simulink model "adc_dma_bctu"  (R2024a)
settings: Solver=FixedStepAuto  StartTime=0.0  StopTime=10.0  FixedStep=0.001  RelTol=1e-3  EnableMultiTasking=on
PreLoadFcn:
  | % NXP_MBDT_S32K3 callback: DO NOT REMOVE
  | mbd_s32k3.common.nxp.model_callbacks.preLoadFcn();
PostLoadFcn:
  | % NXP_MBDT_S32K3 callback: DO NOT REMOVE
  | mbd_s32k3.common.nxp.model_callbacks.postLoadFcn();
InitFcn:
  | % NXP_MBDT_S32K3 callback: DO NOT REMOVE
  | mbd_s32k3.common.nxp.model_callbacks.initFcn();
libraries: mbd_s32k3_io_library x18, mbd_s32k3_isr_library x4, mbd_s32k3_cdd_library x4, mbd_s32k3_utility_library x1, simulink x1

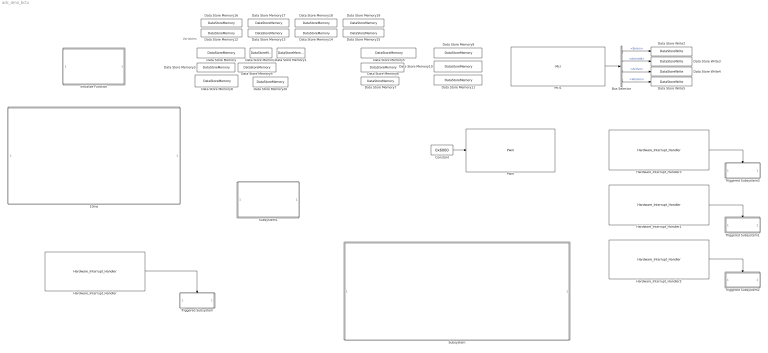
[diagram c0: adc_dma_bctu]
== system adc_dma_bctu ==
  note: Variables
  10ms : Subsystem  TreatAsAtomicUnit=on  SystemSampleTime=0.01
  Bus Selector : BusSelector  Commented=on  OutputSignals=Errors,ActiveId,Active,Version
  Constant : Constant  Commented=on  Value=0x6000
  Data Store Memory : DataStoreMemory  DataStoreName=Adc1_Group0_ResoultBuffer  WriteAfterWriteMsg=warning  ShowAdditionalParam=off  OutDataTypeStr=uint16
  Data Store Memory1 : DataStoreMemory  DataStoreName=GroupStatus  WriteAfterWriteMsg=warning  ShowAdditionalParam=off  OutDataTypeStr=uint32
  Data Store Memory10 : DataStoreMemory  DataStoreName=Bctu_NDataFlag  WriteAfterWriteMsg=warning  ShowAdditionalParam=off  OutDataTypeStr=boolean
  Data Store Memory11 : DataStoreMemory  DataStoreName=Bctu_OvrDataFlag  WriteAfterWriteMsg=warning  ShowAdditionalParam=off  OutDataTypeStr=boolean
  Data Store Memory12 : DataStoreMemory  DataStoreName=Errors_Instance  ReadBeforeWriteMsg=warning  WriteAfterWriteMsg=warning  WriteAfterReadMsg=warning  ShowAdditionalParam=off  OutDataTypeStr=uint32
  Data Store Memory13 : DataStoreMemory  DataStoreName=ActiveId_Instance  ReadBeforeWriteMsg=warning  WriteAfterWriteMsg=warning  WriteAfterReadMsg=warning  ShowAdditionalParam=off  OutDataTypeStr=uint8
  Data Store Memory14 : DataStoreMemory  DataStoreName=Active_Instance  ReadBeforeWriteMsg=warning  WriteAfterWriteMsg=warning  WriteAfterReadMsg=warning  ShowAdditionalParam=off  OutDataTypeStr=boolean
  Data Store Memory15 : DataStoreMemory  DataStoreName=Version_Instance  ReadBeforeWriteMsg=warning  WriteAfterWriteMsg=warning  WriteAfterReadMsg=warning  ShowAdditionalParam=off  OutDataTypeStr=uint8
  Data Store Memory16 : DataStoreMemory  DataStoreName=ChannelState  ReadBeforeWriteMsg=warning  WriteAfterWriteMsg=warning  WriteAfterReadMsg=warning  InitialValue=Mcl_DmaChannelStateType.MCL_DMA_CH_RESET_STATE  ShowAdditionalParam=off  OutDataTypeStr=Enum: Mcl_DmaChannelStateType
  Data Store Memory17 : DataStoreMemory  DataStoreName=Error_Channel  ReadBeforeWriteMsg=warning  WriteAfterWriteMsg=warning  WriteAfterReadMsg=warning  ShowAdditionalParam=off  OutDataTypeStr=uint32
  Data Store Memory18 : DataStoreMemory  DataStoreName=Active_Channel  ReadBeforeWriteMsg=warning  WriteAfterWriteMsg=warning  WriteAfterReadMsg=warning  ShowAdditionalParam=off  OutDataTypeStr=boolean
  Data Store Memory19 : DataStoreMemory  DataStoreName=Done_Channel  ReadBeforeWriteMsg=warning  WriteAfterWriteMsg=warning  WriteAfterReadMsg=warning  ShowAdditionalParam=off  OutDataTypeStr=boolean
  Data Store Memory2 : DataStoreMemory  DataStoreName=ADC_POT0  WriteAfterWriteMsg=warning  ShowAdditionalParam=off  OutDataTypeStr=uint16
  Data Store Memory20 : DataStoreMemory  DataStoreName=Adc1_ChansArray  WriteAfterWriteMsg=warning  ShowAdditionalParam=off  OutDataTypeStr=uint16
  Data Store Memory3 : DataStoreMemory  DataStoreName=Adc1_ReadStatus  WriteAfterWriteMsg=warning  ShowAdditionalParam=off  OutDataTypeStr=uint32
  Data Store Memory4 : DataStoreMemory  DataStoreName=Adc1_BufReadStatus  WriteAfterWriteMsg=warning  ShowAdditionalParam=off  OutDataTypeStr=uint32
  Data Store Memory5 : DataStoreMemory  DataStoreName=Adc0_Group0_ResoulBuffer  WriteAfterWriteMsg=warning  ShowAdditionalParam=off  OutDataTypeStr=uint16
  Data Store Memory6 : DataStoreMemory  DataStoreName=ADC_BCTU_Result  WriteAfterWriteMsg=warning  ShowAdditionalParam=off  OutDataTypeStr=uint16
  Data Store Memory7 : DataStoreMemory  DataStoreName=Adc0_ReadStatus  WriteAfterWriteMsg=warning  ShowAdditionalParam=off  OutDataTypeStr=uint32
  Data Store Memory8 : DataStoreMemory  DataStoreName=Calibration_ADC1_Status  WriteAfterWriteMsg=warning  ShowAdditionalParam=off  OutDataTypeStr=uint8
  Data Store Memory9 : DataStoreMemory  DataStoreName=Bctu_TriggerFlag  WriteAfterWriteMsg=warning  ShowAdditionalParam=off  OutDataTypeStr=boolean
  Data Store Write2 : DataStoreWrite  Commented=on  DataStoreName=Errors_Instance  IndexOptions=Index vector (dialog)  Indices=1  OutputSizes=1
  Data Store Write3 : DataStoreWrite  Commented=on  DataStoreName=ActiveId_Instance  IndexOptions=Index vector (dialog)  Indices=1  OutputSizes=1
  Data Store Write4 : DataStoreWrite  Commented=on  DataStoreName=Active_Instance  IndexOptions=Index vector (dialog)  Indices=1  OutputSizes=1
  Data Store Write5 : DataStoreWrite  Commented=on  DataStoreName=Version_Instance  IndexOptions=Index vector (dialog)  Indices=1  OutputSizes=1
  Hardware_Interrupt_Handler : mbd_s32k3_isr_library/Hardware_Interrupt_Handler  Priority=2  blockCbk=0  irqGroup=Adc  irqHandlers=Adc_Adc1Group0_Callback  irqSim=off  text=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
  Hardware_Interrupt_Handler1 : mbd_s32k3_isr_library/Hardware_Interrupt_Handler  Priority=2  Commented=on  blockCbk=0  irqGroup=Adc  irqHandlers=Bctu_NewData_Cb  irqSim=off  text=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
  Hardware_Interrupt_Handler2 : mbd_s32k3_isr_library/Hardware_Interrupt_Handler  Priority=2  Commented=on  blockCbk=0  irqGroup=Adc  irqHandlers=Bctu_OverrunData_Cb  irqSim=off  text=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
  Hardware_Interrupt_Handler3 : mbd_s32k3_isr_library/Hardware_Interrupt_Handler  Priority=2  Commented=on  blockCbk=0  irqGroup=Adc  irqHandlers=Bctu_Trg_Cb  irqSim=off  text=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
  Initialize Function : Subsystem  TreatAsAtomicUnit=on
  Mcl1 : mbd_s32k3_cdd_library/Mcl  Commented=on  api_func=Mcl_GetDmaInstanceStatus  logicInput=LCU_LOGIC_INPUT_0  logicOutput=LCU_LOGIC_OUTPUT_0  logicInstance=LCU_LOGIC_INSTANCE_0  emiosInstance=EMIOS_2  ftmInstance=FTM0  logicChannel=EMIOS_2_EMIOS_0_MasteBus0  prescalerType=MCL_EMIOS_PRESCALER  dmaLogicInstance=DMA_LOGIC_INST_0  dmaLogicChannel=DMA_LOGIC_CH_0  dmaInstanceCommandType=MCL_DMA_INST_STOP  dmaChannelCommandType=MCL_DMA_CH_START_REQUEST  dmaScatterGatherElement=DMA_LOGIC_CH_0_SGA_ELEMENT_0  dmaChannelInfo=MCL_DMA_CH_GET_SOURCE_ADDRESS  text=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
  Pwm : mbd_s32k3_io_library/Pwm  Commented=on  api_func=Pwm_SetDutyCycle  channel=PwmChannel_0  notification=PWM_RISING_EDGE  moduleId=PWM_EMIOS_INSTANCE_2  prescalerType=PWM_PRIMARY_PRESCALER  fault=PWM_FLEXPWM_0_FAULT_INPUT_0  text=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
  Subsystem : Subsystem  Commented=on  TreatAsAtomicUnit=on  SystemSampleTime=0.001
  Subsystem1 : Subsystem  Commented=on  TreatAsAtomicUnit=on  SystemSampleTime=0.001
  Triggered Subsystem : Subsystem  TreatAsAtomicUnit=on
  Triggered Subsystem1 : Subsystem  Commented=on  TreatAsAtomicUnit=on
  Triggered Subsystem2 : Subsystem  Commented=on  TreatAsAtomicUnit=on
  Triggered Subsystem3 : Subsystem  Commented=on  TreatAsAtomicUnit=on
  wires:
  Constant/1 -> Pwm/1
  Hardware_Interrupt_Handler/1 -> Triggered Subsystem/Trigger
  Hardware_Interrupt_Handler1/1 -> Triggered Subsystem1/Trigger
  Hardware_Interrupt_Handler2/1 -> Triggered Subsystem2/Trigger
  Hardware_Interrupt_Handler3/1 -> Triggered Subsystem3/Trigger
  Bus Selector/2 -> Data Store Write3/1  "<ActiveId>"
  Bus Selector/3 -> Data Store Write4/1  "<Active>"
  Bus Selector/4 -> Data Store Write5/1  "<Version>"
  Mcl1/1 -> Bus Selector/1
  Bus Selector/1 -> Data Store Write2/1  "<Errors>"

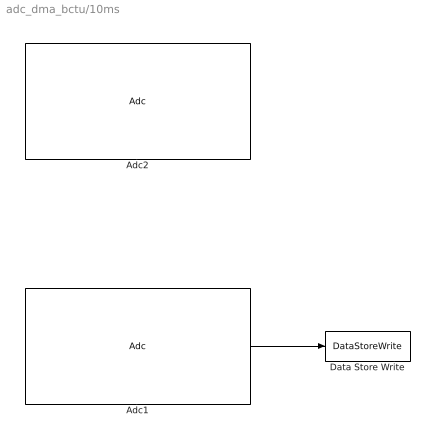
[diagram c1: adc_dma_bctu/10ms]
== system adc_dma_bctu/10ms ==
  Adc1 : mbd_s32k3_io_library/Adc  Priority=2  api_func=Adc_GetGroupStatus  hw_unit=AdcHwUnit_1  group=Adc1Group_0  channel=Adc1_POT_0  threshold_control=No ADC threshold control configured  power_state=ADC_FULL_POWER  ctu_unit=BctuHwUnit_0  ctu_trigger=AdcHwTrigger_0  ctu_fifo_idx=BctuResultFifos_0  text=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
  Adc2 : mbd_s32k3_io_library/Adc  Priority=1  api_func=Adc_StartGroupConversion  hw_unit=AdcHwUnit_1  group=Adc1Group_0  channel=Adc1_POT_0  threshold_control=No ADC threshold control configured  power_state=ADC_FULL_POWER  ctu_unit=BctuHwUnit_0  ctu_trigger=AdcHwTrigger_0  ctu_fifo_idx=BctuResultFifos_0  text=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
  Data Store Write : DataStoreWrite  DataStoreName=GroupStatus  IndexOptions=Index vector (dialog)  Indices=1  OutputSizes=1
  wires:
  Adc1/1 -> Data Store Write/1

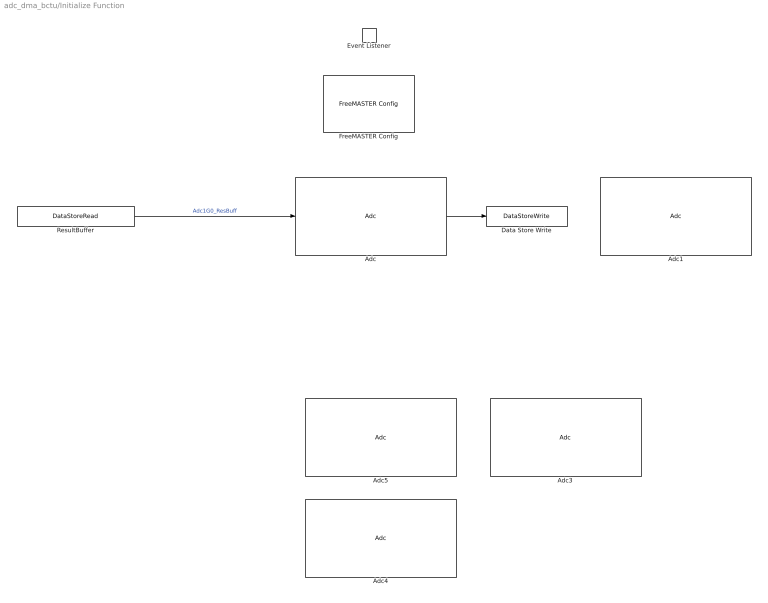
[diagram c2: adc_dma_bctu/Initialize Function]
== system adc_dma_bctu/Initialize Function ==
  Adc : mbd_s32k3_io_library/Adc  Priority=0  api_func=Adc_SetupResultBuffer  hw_unit=AdcHwUnit_1  group=Adc1Group_0  channel=Adc1_POT_0  threshold_control=No ADC threshold control configured  power_state=ADC_FULL_POWER  ctu_unit=BctuHwUnit_0  ctu_trigger=AdcHwTrigger_0  ctu_fifo_idx=BctuResultFifos_0  text=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
  Adc1 : mbd_s32k3_io_library/Adc  api_func=Adc_EnableGroupNotification  hw_unit=AdcHwUnit_1  group=Adc1Group_0  channel=Adc1_POT_0  threshold_control=No ADC threshold control configured  power_state=ADC_FULL_POWER  ctu_unit=BctuHwUnit_0  ctu_trigger=AdcHwTrigger_0  ctu_fifo_idx=BctuResultFifos_0  text=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
  Adc3 : mbd_s32k3_io_library/Adc  Commented=on  api_func=Adc_EnableHardwareTrigger  hw_unit=AdcHwUnit_1  group=Adc1Group_0  channel=Adc1_POT_0  threshold_control=No ADC threshold control configured  power_state=ADC_FULL_POWER  ctu_unit=BctuHwUnit_0  ctu_trigger=AdcHwTrigger_0  ctu_fifo_idx=BctuResultFifos_0  text=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
  Adc4 : mbd_s32k3_io_library/Adc  Priority=1  Commented=on  api_func=Adc_EnableCtuControlMode  hw_unit=AdcHwUnit_1  group=Adc1Group_0  channel=Adc1_POT_0  threshold_control=No ADC threshold control configured  power_state=ADC_FULL_POWER  ctu_unit=BctuHwUnit_0  ctu_trigger=AdcHwTrigger_0  ctu_fifo_idx=BctuResultFifos_0  text=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
  Adc5 : mbd_s32k3_io_library/Adc  Commented=on  api_func=Adc_CtuEnableHwTrigger  hw_unit=AdcHwUnit_1  group=Adc1Group_0  channel=Adc1_POT_0  threshold_control=No ADC threshold control configured  power_state=ADC_FULL_POWER  ctu_unit=BctuHwUnit_0  ctu_trigger=AdcHwTrigger_0  ctu_fifo_idx=BctuResultFifos_0  text=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
  Data Store Write : DataStoreWrite  DataStoreName=Adc1_BufReadStatus  IndexOptions=Index vector (dialog)  Indices=1  OutputSizes=1
  Event Listener : EventListener  DisableCoverage=on  EventName=reset
  FreeMASTER Config : mbd_s32k3_utility_library/FreeMASTER blocks/FreeMASTER Config  connection_type=Serial  instance=LPUART_13  baudrate=115200  isr_prio=0  cantxid=0x7aa  cantxidext=on  cantxobj=5  canrxid=0x7aa  canrxidext=on  canrxobj=5  mode=Short Interrupt  scope_use=1  scope_max_vars=8  automatic_buff_size=on  buff_size=255  default_rfifo_size=on  rfifo_size=32
  ResultBuffer : DataStoreRead  Priority=1  DataStoreName=Adc1_Group0_ResoultBuffer  IndexOptions=Index vector (dialog)  Indices=1  OutputSizes=1
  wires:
  Adc/1 -> Data Store Write/1
  ResultBuffer/1 -> Adc/1  "Adc1G0_ResBuff"

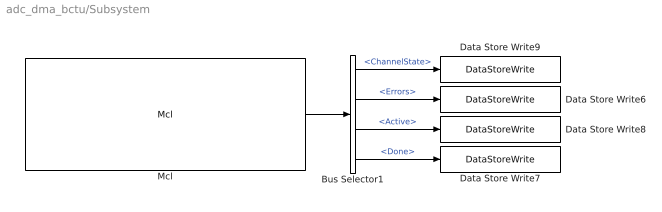
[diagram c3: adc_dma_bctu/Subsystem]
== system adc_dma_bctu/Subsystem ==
  Bus Selector1 : BusSelector  OutputSignals=ChannelState,Errors,Active,Done
  Data Store Write6 : DataStoreWrite  DataStoreName=Error_Channel  IndexOptions=Index vector (dialog)  Indices=1  OutputSizes=1
  Data Store Write7 : DataStoreWrite  DataStoreName=Done_Channel  IndexOptions=Index vector (dialog)  Indices=1  OutputSizes=1
  Data Store Write8 : DataStoreWrite  DataStoreName=Active_Channel  IndexOptions=Index vector (dialog)  Indices=1  OutputSizes=1
  Data Store Write9 : DataStoreWrite  DataStoreName=ChannelState  IndexOptions=Index vector (dialog)  Indices=1  OutputSizes=1
  Mcl : mbd_s32k3_cdd_library/Mcl  api_func=Mcl_GetDmaChannelStatus  logicInput=LCU_LOGIC_INPUT_0  logicOutput=LCU_LOGIC_OUTPUT_0  logicInstance=LCU_LOGIC_INSTANCE_0  emiosInstance=EMIOS_2  ftmInstance=FTM0  logicChannel=EMIOS_2_EMIOS_0_MasteBus0  prescalerType=MCL_EMIOS_PRESCALER  dmaLogicInstance=DMA_LOGIC_INST_0  dmaLogicChannel=DMA_LOGIC_CH_0  dmaInstanceCommandType=MCL_DMA_INST_STOP  dmaChannelCommandType=MCL_DMA_CH_START_REQUEST  dmaScatterGatherElement=DMA_LOGIC_CH_0_SGA_ELEMENT_0  dmaChannelInfo=MCL_DMA_CH_GET_SOURCE_ADDRESS  text=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
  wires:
  Bus Selector1/3 -> Data Store Write8/1  "<Active>"
  Mcl/1 -> Bus Selector1/1
  Bus Selector1/1 -> Data Store Write9/1  "<ChannelState>"
  Bus Selector1/4 -> Data Store Write7/1  "<Done>"
  Bus Selector1/2 -> Data Store Write6/1  "<Errors>"

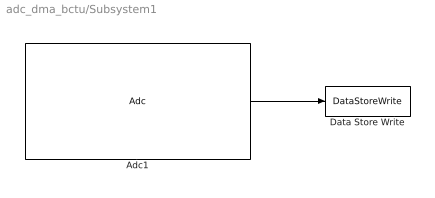
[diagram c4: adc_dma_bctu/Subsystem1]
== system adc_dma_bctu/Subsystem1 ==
  Adc1 : mbd_s32k3_io_library/Adc  Priority=2  api_func=Adc_GetGroupStatus  hw_unit=AdcHwUnit_1  group=Adc1Group_0  channel=Adc1_POT_0  threshold_control=No ADC threshold control configured  power_state=ADC_FULL_POWER  ctu_unit=BctuHwUnit_0  ctu_trigger=AdcHwTrigger_0  ctu_fifo_idx=BctuResultFifos_0  text=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
  Data Store Write : DataStoreWrite  DataStoreName=GroupStatus  IndexOptions=Index vector (dialog)  Indices=1  OutputSizes=1
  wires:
  Adc1/1 -> Data Store Write/1

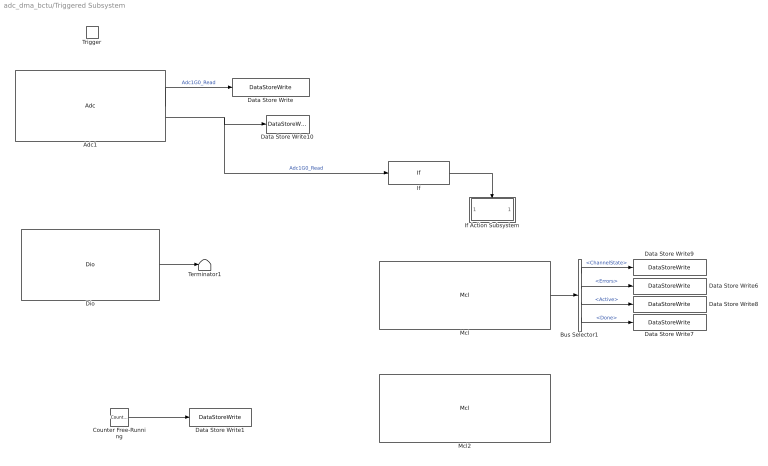
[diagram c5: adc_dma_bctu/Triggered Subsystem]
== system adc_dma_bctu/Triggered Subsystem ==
  Trigger : TriggerPort  TriggerType=function-call  VariantControl=(inherit)
  Adc1 : mbd_s32k3_io_library/Adc  api_func=Adc_ReadGroup  hw_unit=AdcHwUnit_1  group=Adc1Group_0  channel=Adc1_POT_0  threshold_control=No ADC threshold control configured  power_state=ADC_FULL_POWER  ctu_unit=BctuHwUnit_0  ctu_trigger=AdcHwTrigger_0  ctu_fifo_idx=BctuResultFifos_0  text=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
  Bus Selector1 : BusSelector  OutputSignals=ChannelState,Errors,Active,Done
  Counter Free-Running : simulink/Sources/Counter Free-Running  Commented=on  NumBits=16  tsamp=-1
  Data Store Write : DataStoreWrite  DataStoreName=Adc1_ReadStatus  IndexOptions=Index vector (dialog)  Indices=1  OutputSizes=1
  Data Store Write1 : DataStoreWrite  Commented=on  DataStoreName=Adc1_ChansArray  IndexOptions=Index vector (dialog)  Indices=1  OutputSizes=1
  Data Store Write10 : DataStoreWrite  DataStoreName=ADC_POT0  IndexOptions=Index vector (dialog)  Indices=1  OutputSizes=1
  Data Store Write6 : DataStoreWrite  DataStoreName=Error_Channel  IndexOptions=Index vector (dialog)  Indices=1  OutputSizes=1
  Data Store Write7 : DataStoreWrite  DataStoreName=Done_Channel  IndexOptions=Index vector (dialog)  Indices=1  OutputSizes=1
  Data Store Write8 : DataStoreWrite  DataStoreName=Active_Channel  IndexOptions=Index vector (dialog)  Indices=1  OutputSizes=1
  Data Store Write9 : DataStoreWrite  DataStoreName=ChannelState  IndexOptions=Index vector (dialog)  Indices=1  OutputSizes=1
  Dio : mbd_s32k3_io_library/Dio  api_func=Dio_FlipChannel  channel=RGBLED0_GREEN  channel_group=No channel groups configured  port=PTF_H  gpioSim=off  text=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
  If : If  IfExpression=u1 > 10000
  If Action Subsystem : Subsystem  TreatAsAtomicUnit=on
  Mcl : mbd_s32k3_cdd_library/Mcl  api_func=Mcl_GetDmaChannelStatus  logicInput=LCU_LOGIC_INPUT_0  logicOutput=LCU_LOGIC_OUTPUT_0  logicInstance=LCU_LOGIC_INSTANCE_0  emiosInstance=EMIOS_2  ftmInstance=FTM0  logicChannel=EMIOS_2_EMIOS_0_MasteBus0  prescalerType=MCL_EMIOS_PRESCALER  dmaLogicInstance=DMA_LOGIC_INST_0  dmaLogicChannel=DMA_LOGIC_CH_0  dmaInstanceCommandType=MCL_DMA_INST_STOP  dmaChannelCommandType=MCL_DMA_CH_START_REQUEST  dmaScatterGatherElement=DMA_LOGIC_CH_0_SGA_ELEMENT_0  dmaChannelInfo=MCL_DMA_CH_GET_SOURCE_ADDRESS  text=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
  Mcl2 : mbd_s32k3_cdd_library/Mcl  api_func=Mcl_SetDmaChannelCommand  logicInput=LCU_LOGIC_INPUT_0  logicOutput=LCU_LOGIC_OUTPUT_0  logicInstance=LCU_LOGIC_INSTANCE_0  emiosInstance=EMIOS_2  ftmInstance=FTM0  logicChannel=EMIOS_2_EMIOS_0_MasteBus0  prescalerType=MCL_EMIOS_PRESCALER  dmaLogicInstance=DMA_LOGIC_INST_0  dmaLogicChannel=DMA_LOGIC_CH_0  dmaInstanceCommandType=MCL_DMA_INST_STOP  dmaChannelCommandType=MCL_DMA_CH_ACK_DONE  dmaScatterGatherElement=DMA_LOGIC_CH_0_SGA_ELEMENT_0  dmaChannelInfo=MCL_DMA_CH_GET_SOURCE_ADDRESS  text=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
  Terminator1 : Terminator
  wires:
  Dio/1 -> Terminator1/1
  Adc1/2 -> If/1, Data Store Write10/1  "Adc1G0_Read"
  Adc1/1 -> Data Store Write/1  "Adc1G0_Read"
  Bus Selector1/2 -> Data Store Write6/1  "<Errors>"
  Bus Selector1/1 -> Data Store Write9/1  "<ChannelState>"
  Bus Selector1/3 -> Data Store Write8/1  "<Active>"
  Bus Selector1/4 -> Data Store Write7/1  "<Done>"
  Mcl/1 -> Bus Selector1/1
  If/1 -> If Action Subsystem/Action
  Counter Free-Running/1 -> Data Store Write1/1

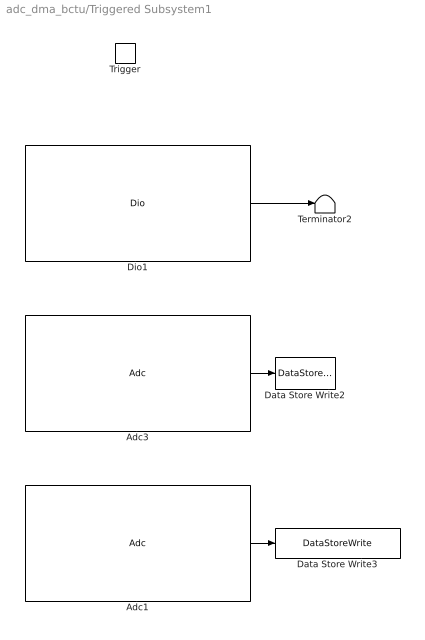
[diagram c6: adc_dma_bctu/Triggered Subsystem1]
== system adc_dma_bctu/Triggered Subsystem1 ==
  Trigger : TriggerPort  TriggerType=function-call  VariantControl=(inherit)
  Adc1 : mbd_s32k3_io_library/Adc  Commented=on  api_func=Adc_CtuReadConvResult  hw_unit=AdcHwUnit_1  group=Adc1Group_0  channel=Adc1_POT_0  threshold_control=No ADC threshold control configured  power_state=ADC_FULL_POWER  ctu_unit=BctuHwUnit_0  ctu_trigger=AdcHwTrigger_0  ctu_fifo_idx=BctuResultFifos_0  text=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
  Adc3 : mbd_s32k3_io_library/Adc  api_func=Adc_CtuReadConvData  hw_unit=AdcHwUnit_1  group=Adc1Group_0  channel=Adc1_POT_0  threshold_control=No ADC threshold control configured  power_state=ADC_FULL_POWER  ctu_unit=BctuHwUnit_0  ctu_trigger=AdcHwTrigger_0  ctu_fifo_idx=BctuResultFifos_0  text=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
  Data Store Write2 : DataStoreWrite  DataStoreName=Adc1_ChansArray  IndexOptions=Index vector (dialog)  Indices=1  OutputSizes=1
  Data Store Write3 : DataStoreWrite  Commented=on  DataStoreName=ADC_BCTU_Result  IndexOptions=Index vector (dialog)  Indices=1  OutputSizes=1
  Dio1 : mbd_s32k3_io_library/Dio  api_func=Dio_FlipChannel  channel=RGBLED0_GREEN  channel_group=No channel groups configured  port=PTF_H  gpioSim=off  text=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
  Terminator2 : Terminator
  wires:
  Adc3/1 -> Data Store Write2/1
  Adc1/1 -> Data Store Write3/1
  Dio1/1 -> Terminator2/1

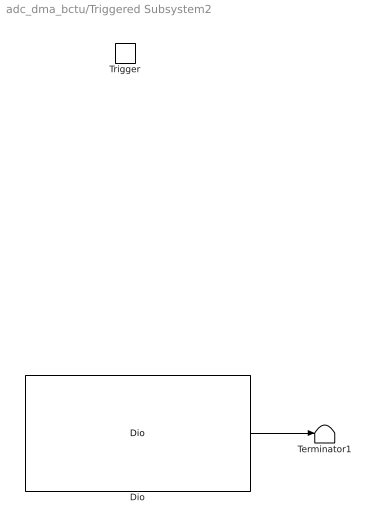
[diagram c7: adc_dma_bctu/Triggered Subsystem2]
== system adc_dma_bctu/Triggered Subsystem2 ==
  Trigger : TriggerPort  TriggerType=function-call  VariantControl=(inherit)
  Dio : mbd_s32k3_io_library/Dio  api_func=Dio_FlipChannel  channel=RGBLED0_RED  channel_group=No channel groups configured  port=PTF_H  gpioSim=off  text=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
  Terminator1 : Terminator
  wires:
  Dio/1 -> Terminator1/1

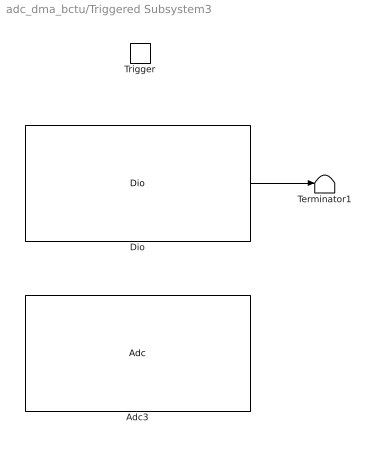
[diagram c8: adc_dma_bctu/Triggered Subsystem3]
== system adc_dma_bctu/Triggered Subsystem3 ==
  Trigger : TriggerPort  TriggerType=function-call  VariantControl=(inherit)
  Adc3 : mbd_s32k3_io_library/Adc  Commented=on  api_func=Adc_CtuStartConversion  hw_unit=AdcHwUnit_1  group=Adc1Group_0  channel=Adc1_POT_0  threshold_control=No ADC threshold control configured  power_state=ADC_FULL_POWER  ctu_unit=BctuHwUnit_0  ctu_trigger=AdcHwTrigger_0  ctu_fifo_idx=BctuResultFifos_0  text=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
  Dio : mbd_s32k3_io_library/Dio  api_func=Dio_FlipChannel  channel=RGBLED0_BLUE  channel_group=No channel groups configured  port=PTF_H  gpioSim=off  text=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
  Terminator1 : Terminator
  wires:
  Dio/1 -> Terminator1/1

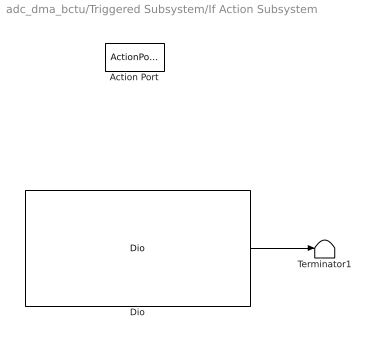
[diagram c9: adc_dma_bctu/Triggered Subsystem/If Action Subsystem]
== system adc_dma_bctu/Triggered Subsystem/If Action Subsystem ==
  Action Port : ActionPort  ActionPortLabel=if(u1 > 10000)
  Dio : mbd_s32k3_io_library/Dio  api_func=Dio_FlipChannel  channel=RGBLED1_BLUE  channel_group=No channel groups configured  port=PTF_H  gpioSim=off  text=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
  Terminator1 : Terminator
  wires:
  Dio/1 -> Terminator1/1
